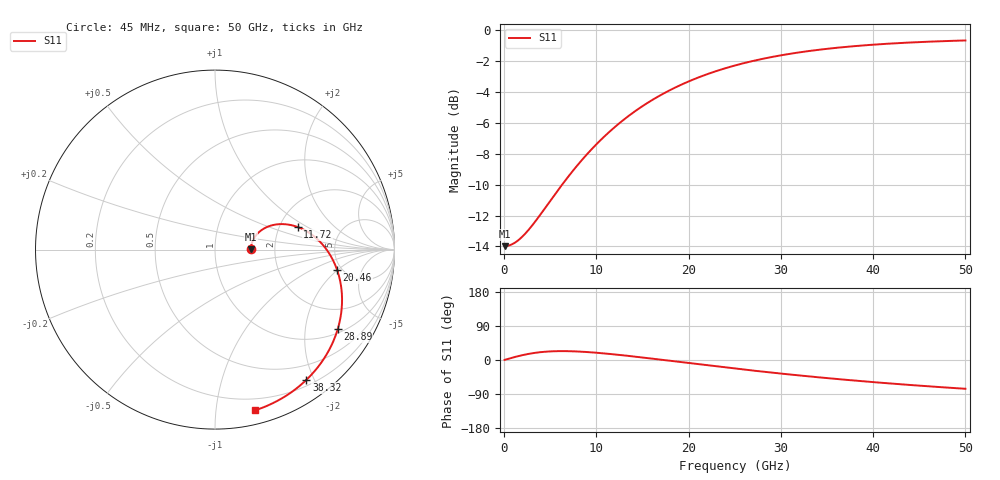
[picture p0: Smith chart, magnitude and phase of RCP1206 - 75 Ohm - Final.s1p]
!Vishay Electro-Films Inc.
!RCP Family
!Case Size 1206
!Assembly Style Surface Mount
!11/2/2015
!efi@vishay.com
# GHz S MA R 50
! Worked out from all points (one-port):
!   801 points, 45 MHz to 50 GHz, reference 50 ohm
!   lowest |S11| = -14.0 dB at 45 MHz (marker M1), VSWR 1.50, Z = 75 + j0.173 ohm
!   |S11| at or under -10 dB: start of sweep to 6.289 GHz
!   S11 on the Smith chart (normalised r, x): 45 MHz: 1.50, +0.00; 11.72 GHz: 2.51, +0.82; 20.46 GHz: 4.56, -1.97; 28.89 GHz: 1.13, -2.99; 38.32 GHz: 0.28, -1.89; 50 GHz: 0.11, -1.28
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0.045  0.2 0.3
1.106544  0.2048 7.6
2.230531  0.2187 14.1
3.0423  0.2335 17.8
4.166288  0.2588 21.2
6.289375  0.3162 23.5
7.663138  0.3567 22.8
9.0369  0.3979 20.9
10.34822  0.437 18.4
11.72198  0.4771 15.3
12.53375  0.5002 13.3
13.96996  0.5396 9.4
15.46861  0.5785 5.2
17.15459  0.6193 0.3
18.77812  0.6554 -4.5
20.46411  0.6897 -9.5
22.71208  0.7303 -16.0
25.0225  0.7663 -22.6
26.89581  0.7915 -27.7
28.89401  0.8149 -33.0
31.26687  0.8383 -39.0
34.38906  0.8631 -46.4
37.51125  0.8823 -53.2
38.32302  0.8865 -54.9
41.0081  0.8985 -60.3
43.75563  0.9081 -65.5
46.87781  0.9166 -70.9
50  0.9229 -75.9
